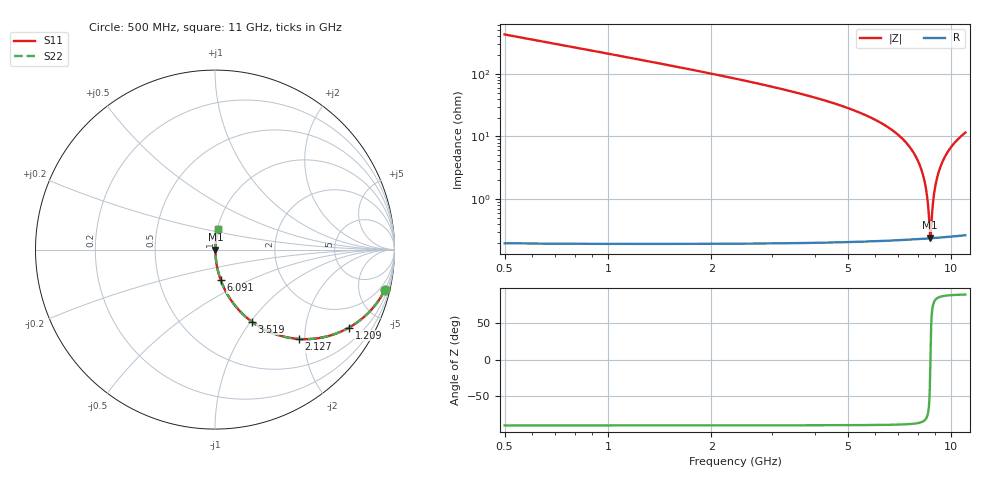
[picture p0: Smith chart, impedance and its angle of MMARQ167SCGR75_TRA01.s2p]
! MMARQ167SCGR75_TRA01  S-PARAMETER MODEL  ( General Type )
! Model Generated by TAIYO YUDEN Corporation (http://www.ty-top.com)
! Version 1.0
! TAIYO YUDEN Control No. 160201
! Copyright(c) 2016 TAIYO YUDEN CO.,LTD. All Rights Reserved.
! Product Description (link to TY-COMPAS)
! https://ds.yuden.co.jp/TYCOMPAS/or/detail?pn=MMARQ167SCGR75BTRA01&u=M
! Products Name : Multilayer Ceramic Capacitors
! Characteristics :
!  Capacitance : 0.75 pF , Rated Voltage : 250V , TCC : CG / C0G
!  Case Size : 1.6 x 0.8 / 0.063 x 0.031 [mm/inch] , Thickness : 0.7 / 0.028 [mm/inch]
!  (Conditions: Temperature = 25 degC , DC Bias Current/Voltage = 0A / 0V)
! External Node Assignments :
!  1  o---| |---o  2
! GND o---------o GND
! Frequency Range : 500MHz  -  11000MHz  [ 401 STEP ]
# MHz S RI R 50
! Freq[MHz].  S11 Real  S11 Imag  S21 Real  S21 Imag  S12 Real  S12 Imag  S22 Real  S22 Imag
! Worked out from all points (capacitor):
!   401 points, 500 MHz to 11 GHz, reference 50 ohm
!   read as one part in series: C = 751 fF near 552.5 MHz
!   lowest |Z| = 244 mohm at 8.69 GHz (marker M1)
!   series resonance near 8.699 GHz, so ESL is about 450 pH
!   S11 on the Smith chart (normalised r, x): 500 MHz: 1.00, -8.45; 1.209 GHz: 1.00, -3.44; 2.127 GHz: 1.00, -1.87; 3.519 GHz: 1.00, -1.01; 6.091 GHz: 1.00, -0.35; 11 GHz: 1.01, +0.23
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500  0.9469 -0.224  0.0531 0.224  0.0531 0.224  0.9469 -0.224
841.25  0.8616 -0.345  0.1384 0.345  0.1384 0.345  0.8616 -0.345
1208.75  0.7472 -0.4341  0.2528 0.4341  0.2528 0.4341  0.7472 -0.4341
2127.5  0.4676 -0.4979  0.5324 0.4979  0.5324 0.4979  0.4676 -0.4979
2258.75  0.434 -0.4945  0.566 0.4945  0.566 0.4945  0.434 -0.4945
3518.75  0.2035 -0.4006  0.7965 0.4006  0.7965 0.4006  0.2035 -0.4006
4017.5  0.1483 -0.3529  0.8517 0.3529  0.8517 0.3529  0.1483 -0.3529
5750  0.0432 -0.1983  0.9568 0.1983  0.9568 0.1983  0.0432 -0.1983
6091.25  0.0325 -0.1713  0.9675 0.1713  0.9675 0.1713  0.0325 -0.1713
7508.75  0.00738 -0.0713  0.9926 0.0713  0.9926 0.0713  0.00738 -0.0713
7981.25  0.00406 -0.0418  0.9959 0.0418  0.9959 0.0418  0.00406 -0.0418
8322.5  0.0028 -0.0215  0.9972 0.0215  0.9972 0.0215  0.0028 -0.0215
8506.25  0.00248 -0.0109  0.9975 0.0109  0.9975 0.0109  0.00248 -0.0109
8585  0.00241 -0.00642  0.9976 0.00642  0.9976 0.00642  0.00241 -0.00642
8663.75  0.00238 -0.00199  0.9976 0.00199  0.9976 0.00199  0.00238 -0.00199
8690  0.00238 -0.00052  0.9976 0.00052  0.9976 0.00052  0.00238 -0.00052
8742.5  0.00239 0.0024  0.9976 -0.0024  0.9976 -0.0024  0.00239 0.0024
8847.5  0.00246 0.00819  0.9975 -0.00819  0.9975 -0.00819  0.00246 0.00819
8952.5  0.0026 0.0139  0.9974 -0.0139  0.9974 -0.0139  0.0026 0.0139
9267.5  0.00339 0.0307  0.9966 -0.0307  0.9966 -0.0307  0.00339 0.0307
9950  0.00679 0.0651  0.9932 -0.0651  0.9932 -0.0651  0.00679 0.0651
11000  0.0157 0.1133  0.9843 -0.1133  0.9843 -0.1133  0.0157 0.1133
